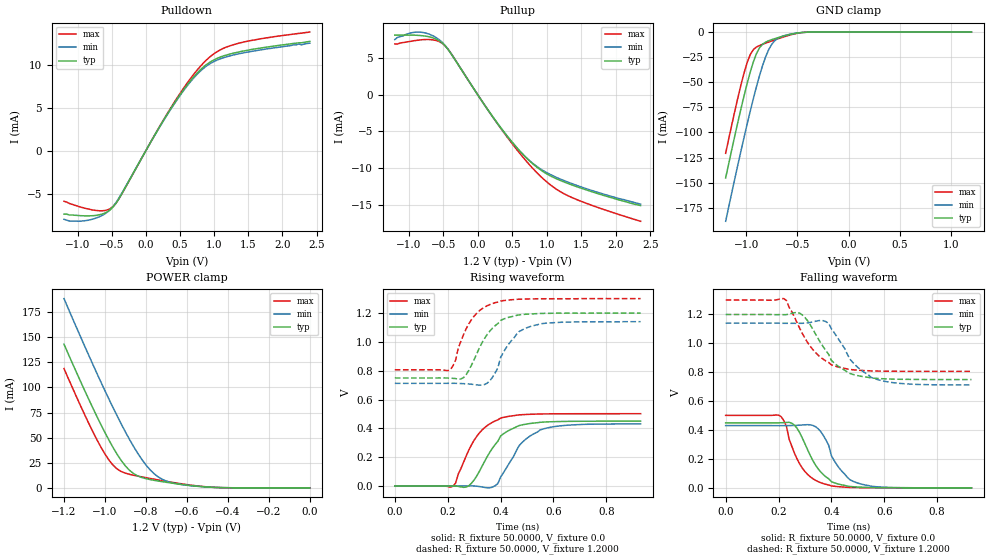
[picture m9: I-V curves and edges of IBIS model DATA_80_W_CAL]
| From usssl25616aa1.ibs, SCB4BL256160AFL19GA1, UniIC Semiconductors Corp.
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|   Model DATA_80_W_CAL
[Model]  DATA_80_W_CAL
Model_type I/O
Polarity   Non-Inverting
Enable   Active-High
Vinl =   0.3800V
Vinh =   0.8200V
Vmeas =  0.6000V
Cref =   5.0000pF
Rref =   50.0000
Vref =   0.6000V
C_comp   1.7430pF   1.7110pF   1.7640pF
[Temperature Range]   25.0000   0.1250k   -40.0000
[Voltage Range]   1.2000V   1.1400V   1.3000V
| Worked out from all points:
|   slope of the pulldown table from 0 to 0.18 V, typ, clamps not added: 72.3 ohm
|   slope of the pullup table from 0 to 0.18 V, typ, clamps not added: 72.5 ohm
|   GND clamp passes 1 mA (typ) near -0.50 V on its own axis
|   POWER clamp passes 1 mA (typ) near -0.51 V on its own axis
|   rising waveform, R_fixture 50.0000, V_fixture 0.0: 20-80 % time 93.1ps typ, 101ps min, 93.2ps max; typ from 0 V to 0.45 V
|   rising waveform, R_fixture 50.0000, V_fixture 1.2000: 20-80 % time 87.8ps typ, 78.5ps min, 77.6ps max; typ from 0.75 V to 1.2 V
|   falling waveform, R_fixture 50.0000, V_fixture 0.0: 20-80 % time 84.5ps typ, 79.2ps min, 73.5ps max; typ from 0.45 V to 0 V
|   falling waveform, R_fixture 50.0000, V_fixture 1.2000: 20-80 % time 102ps typ, 108ps min, 103ps max; typ from 1.2 V to 0.75 V
[Pulldown]
|Voltage   I(typ)   I(min)   I(max)
-1.2V     -7.4mA     -8mA       -5.9mA
-1V       -7.55mA    -8.23mA    -6.47mA
-760mV    -7.573mA   -7.94mA    -6.943mA
-600mV    -7.269mA   -7.364mA   -6.976mA
-480mV    -6.557mA   -6.497mA   -6.508mA
-360mV    -5.125mA   -5.057mA   -5.145mA
400mV     5.32mA     5.244mA    5.423mA
680mV     8.39mA     8.266mA    8.665mA
880mV     9.962mA    9.796mA    10.49mA
1.12V     10.97mA    10.76mA    11.84mA
1.36V     11.47mA    11.26mA    12.49mA
2.4V      12.7mA     12.5mA     13.79mA
[Pullup]
|Voltage   I(typ)   I(min)   I(max)
-1.2V     8.1mA      7.5mA      6.9mA
-1.04V    8.11mA     8.2mA      7.15mA
-840mV    8.05mA     8.51mA     7.44mA
-680mV    7.819mA    8.152mA    7.489mA
-520mV    7.078mA    7.176mA    7.032mA
-400mV    5.766mA    5.809mA    5.8mA
320mV     -4.305mA   -4.359mA   -4.396mA
560mV     -7.129mA   -7.166mA   -7.403mA
800mV     -9.426mA   -9.364mA   -10.05mA
1.08V     -11.18mA   -10.99mA   -12.47mA
1.32V     -12.13mA   -11.95mA   -13.81mA
2.36V     -15.1mA    -14.9mA    -17.23mA
[GND_clamp]
|Voltage   I(typ)   I(min)   I(max)
-1.2V     -145.3mA   -188.5mA   -120.8mA
-1.05V    -76.2mA    -118.2mA   -52.43mA
-990mV    -51.2mA    -91.62mA   -30.39mA
-960mV    -39.9mA    -78.82mA   -22.48mA
-900mV    -21.67mA   -54.7mA    -15mA
-870mV    -15.78mA   -43.66mA   -13.45mA
-810mV    -10.04mA   -24.79mA   -11.07mA
-780mV    -8.658mA   -17.59mA   -9.958mA
-720mV    -6.57mA    -8.545mA   -7.793mA
-630mV    -3.906mA   -3.64mA    -4.741mA
-420mV    -215.4uA   -240.5uA   -235uA
1.2V      1.597nA    22.84nA    1.463nA
[POWER_clamp]
|Voltage   I(typ)   I(min)   I(max)
-1.2V     143mA      188.4mA    118.7mA
-1.1V     97.38mA    141.5mA    73.24mA
-1.04V    71.38mA    114.3mA    48.22mA
-1V       55.04mA    96.69mA    33.64mA
-960mV    40mA       79.65mA    22.42mA
-900mV    21.75mA    55.6mA     14.58mA
-860mV    14.17mA    41.05mA    12.52mA
-800mV    9.133mA    22.79mA    10.12mA
-740mV    6.786mA    10.88mA    7.886mA
-660mV    4.332mA    4.436mA    5.101mA
-520mV    1.103mA    1.063mA    1.274mA
0V        1.597nA    6.003nA    2.16nA
[Ramp]
| variable   typ   min   max
dV/dt_r  0.2701/95.9095p   0.2585/0.1033n   0.3011/86.6477p
dV/dt_f  0.2703/0.1038n   0.2566/0.1098n   0.2963/96.2373p
R_load = 50.0000
[Rising Waveform]
R_fixture= 50.0000
V_fixture= 0.0
V_fixture_min= 0.0
V_fixture_max= 0.0
|time   V(typ)   V(min)   V(max)
0s        0V         0V         0V
220ps     1.302mV    168.3uV    -1.621mV
270ps     -7.188mV   1.265mV    208.8mV
290ps     19.5mV     1.263mV    286mV
330ps     137.1mV    -6.19mV    388.4mV
370ps     264.3mV    -7.032mV   442.8mV
400ps     346.6mV    61.87mV    471.2mV
470ps     419.3mV    279.8mV    493.6mV
550ps     442.3mV    389.4mV    499.9mV
930ps     450.1mV    430.8mV    501.8mV
[Rising Waveform]
R_fixture= 50.0000
V_fixture= 1.2000
V_fixture_min= 1.1400
V_fixture_max= 1.3000
|time   V(typ)   V(min)   V(max)
0s        749.5mV    712.2mV    806.2mV
210ps     748.3mV    712.6mV    807.1mV
260ps     752.1mV    710.1mV    1.05V
300ps     876.7mV    703.9mV    1.178V
350ps     1.053V     714.3mV    1.251V
390ps     1.127V     820.2mV    1.276V
400ps     1.148V     891.5mV    1.283V
470ps     1.187V     1.071V     1.296V
550ps     1.197V     1.125V     1.299V
930ps     1.2V       1.14V      1.3V
[Falling Waveform]
R_fixture= 50.0000
V_fixture= 0.0
V_fixture_min= 0.0
V_fixture_max= 0.0
|time   V(typ)   V(min)   V(max)
0s        450.1mV    430.9mV    501.8mV
210ps     450.5mV    430.6mV    492.6mV
230ps     452.6mV    430.6mV    425.9mV
250ps     447.6mV    431.4mV    289mV
280ps     382.1mV    433.7mV    165.7mV
330ps     188.6mV    432mV      63.22mV
370ps     90.71mV    361.5mV    29.11mV
420ps     29.49mV    161.3mV    9.08mV
500ps     5.41mV     32.78mV    1.58mV
930ps     748nV      7.85uV     0V
[Falling Waveform]
R_fixture= 50.0000
V_fixture= 1.2000
V_fixture_min= 1.1400
V_fixture_max= 1.3000
|time   V(typ)   V(min)   V(max)
0s        1.2V       1.14V      1.3V
220ps     1.199V     1.139V     1.31V
290ps     1.197V     1.139V     1.069V
370ps     974mV      1.157V     889.3mV
390ps     923.2mV    1.138V     867.6mV
420ps     849.8mV    1.049V     839.5mV
480ps     786mV      870.1mV    817.5mV
560ps     759.1mV    758.2mV    809mV
670ps     751.3mV    721.5mV    806.7mV
930ps     749.5mV    712.3mV    806.2mV
